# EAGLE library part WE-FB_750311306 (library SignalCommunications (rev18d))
WE-FB Flyback Transformer suitable for LT3573/ LT3574/ LT3575/ LT3748 Characteristics easy design in solution less external components needed small board space low cost no optocoupler needed! long term reliability voltage control no aging same external parts for different output voltages easy design of custom power supply due to standard circuit and change of transformers and two components for feedback loop Isolation voltage up to 2.5 kV Applications Isolated power design Sensor interfaces Isolated telecom converters Power over Ethernet Details see: http://katalog.we-online.de/en/pbs/WE-FB_Linear? Updated 2014-07-07 2014 (C) Wurth Elektronik
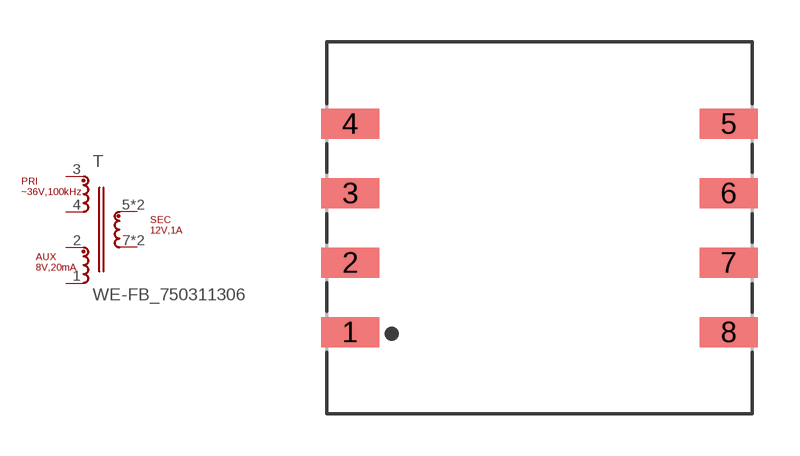
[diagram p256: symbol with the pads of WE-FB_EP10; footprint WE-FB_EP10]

Designator prefix T

## WE-FB_750311306  [WE-FB_EP10]
1  4  pas
2  5  pas
3  1  pas
4  6  pas
5  2  pas
6  2  pas
7  3  pas
8  3  pas

## Footprint WE-FB_EP10 (pad centres in mm)
smd 2.08 x 1.07: 1 -6.78,-3.735; 2 -6.78,-1.245; 3 -6.78,1.245; 4 -6.78,3.735; 5 6.78,3.735; 6 6.78,1.245; 7 6.78,-1.245; 8 6.78,-3.735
